PROGRAM MAIN
(*这这个程序的目的是用于检测EL6022或EL6002模块的好坏,
程序运行后，如果EL2004的1通道灯常量，则代表这个通信模块的2个通道都是好的
1、确保这2个通道的波特率设置都一样，比如9600,n,8,1.改为后reload IO一次，或者64616F6C恢复出厂设置
2、接线正确，232通信要1和5脚交叉连接，3脚直连. 485通信为 2 3短接为+ ，7 8 短接为 - 。
*)
VAR
	master: ModbusRtuMaster_KL6x22B;//EL6022上口
	writearray:ARRAY [1..4] OF WORD;//modsim 03口写操作数组
	readarray:ARRAY [1..4] OF WORD;//modsim 03口读操作数组	
 	state1: INT;
		
	slave: ModbusRtuSlave_KL6x22B;//EL6022下口
	inputs: ARRAY[1..100] OF WORD;
	outputs: ARRAY[1..100] OF WORD;
	memorys: ARRAY[1..100] OF WORD;
	KL2408 AT %Q*: BOOL;
END_VAR

CASE state1 OF 
	0:
		writearray[1]:=writearray[1]+1;
		state1:=1;
	1://03口写操作
			master.WriteRegs(
				UnitID:= 1, 
				Quantity:=4, 
				MBAddr:= 16384, 
				cbLength:= SIZEOF(writearray), 
				pMemoryAddr:= ADR(writearray), 
				Execute:= TRUE, 
				Timeout:= T#500MS, 
				BUSY=> , 
				Error=> , 
				ErrorId=> , 
				cbRead=> );			
				IF NOT master.BUSY THEN
					master.ReadRegs(Execute:= FALSE, );	
					state1:=2;
				END_IF
				
				
	2://03口读操作
			master.ReadRegs(
				UnitID:= 1, 
				Quantity:=4, 
				MBAddr:= 16384, 
				cbLength:= SIZEOF(readarray), 
				pMemoryAddr:= ADR(readarray), 
				Execute:= TRUE, 
				Timeout:= T#500MS, 
				 );	
				IF NOT master.BUSY THEN
					master.ReadRegs(Execute:= FALSE, );	
					state1:=3;
				END_IF		
	3:
		IF writearray[1]=readarray[1]
			THEN KL2408:=TRUE;
				 state1:=0;
			ELSE KL2408:=FALSE;
				state1:=1;
		END_IF
		
END_CASE

slave(
	UnitID:=1 , 
	AdrInputs:=ADR(inputs) , 
	SizeInputBytes:= SIZEOF(inputs), 
	AdrOutputs:= ADR(outputs), 
	SizeOutputBytes:= SIZEOF(outputs), 
	AdrMemory:= ADR(memorys), 
	SizeMemoryBytes:= SIZEOF(memorys), 
	ErrorId=> );

END_PROGRAM
